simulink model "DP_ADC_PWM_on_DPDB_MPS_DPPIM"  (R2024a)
settings: Solver=FixedStepDiscrete  StartTime=0.0  StopTime=inf  FixedStep=10e-6  RelTol=1e-3  EnableMultiTasking=on
model workspace (MAT data in the model file):
  Freq = 100
  Phas = 0
undefined symbols (not defined in the file): a, A0, A2, A8, AD1, AD2, AD3, AD4, AD5, ADC, address, also, AN0, AN1, AN3, AN4, as, B, B0, B5, B6, B8, below, bit, bits, BOR, C6, C7, cause, characters, Code, Communicate, contains, counter, Data, data, dead, default, deviced, disasserted, DS70005399D, dsPIC33AK512MPS506_DPDB_External_v4, dsPIC33AK512MPS506_DPDB_External_v5, dsPIC33CK64MC105, EC, ECIO, ensure, events, Family, faster, Floating, fulll, highest, HS, HS3, I, I2C, I2C1, I2C2, I2C3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
libraries: MCHP_Blockset x10, simulink x1
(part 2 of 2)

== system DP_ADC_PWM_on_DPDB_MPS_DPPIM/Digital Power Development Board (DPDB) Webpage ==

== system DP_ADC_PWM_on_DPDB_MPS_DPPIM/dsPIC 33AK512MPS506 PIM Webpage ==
